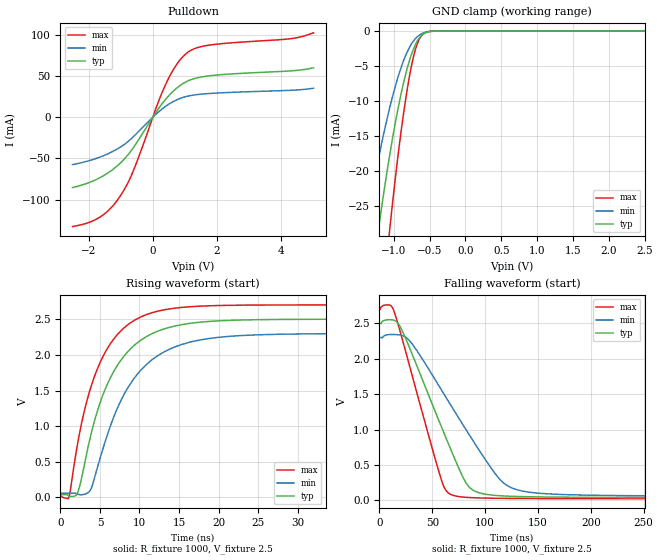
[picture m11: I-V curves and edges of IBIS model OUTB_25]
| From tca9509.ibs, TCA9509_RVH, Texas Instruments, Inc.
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[Model]   OUTB_25
Model_type  Open_drain
Enable   Active-High
Vref =   2.5
Rref =   1350
Cref =   50p
Vmeas =   1.25
| variable   typ   min   max
C_comp   2.86pF   1.87pF   3.29pF
| C_pulldown   2.91pF   2.13pF   4.07pF
| C_tri-state   2.86pF   1.87pF   3.29pF
[Temperature Range]   40   100   -40
| Ambient temperature   25   85   -40
[Voltage range]   2.5   2.3   2.7
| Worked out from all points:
|   slope of the pulldown table from 0 to 0.375 V, typ, clamps not added: 18.2 ohm
|   GND clamp passes 1 mA (typ) near -0.64 V on its own axis
|   rising waveform, R_fixture 1000, V_fixture 2.5: 20-80 % time 5.07ns typ, 5.86ns min, 4.5ns max; typ from 0.04 V to 2.5 V
|   falling waveform, R_fixture 1000, V_fixture 2.5: 20-80 % time 40.3ns typ, 56.6ns min, 29.6ns max; typ from 2.5 V to 0.04 V
[GND Clamp]
| OUTB_25
|   Voltage   I(typ)   I(min)   I(max)
-2.5V     -157.5mA   -111.4mA   -232.4mA
-1.4V     -43.18mA   -28.52mA   -67.74mA
-1.23V    -29.68mA   -19.14mA   -47.05mA
-1.205V   -27.84mA   -17.87mA   -44.2mA
-1.07V    -18.63mA   -11.58mA   -29.8mA
-1.05V    -17.38mA   -10.74mA   -27.82mA
-915mV    -9.842mA   -5.777mA   -15.78mA
-800mV    -4.902mA   -2.742mA   -7.638mA
-715mV    -2.35mA    -1.307mA   -3.298mA
-625mV    -778.3uA   -472.3uA   -845.3uA
-430mV    -20.32uA   -20.58uA   -8.486uA
2.5V      479.8pA    2.008nA    172pA
[Pulldown]
| OUTB_25
|   Voltage   I(typ)   I(min)   I(max)
-2.5V     -85.34mA   -57.53mA   -132.8mA
-1.635V   -73.16mA   -48.24mA   -121mA
-1.31V    -65.26mA   -42.78mA   -110.5mA
-1.01V    -55.58mA   -36.27mA   -95.43mA
-605mV    -36.88mA   -23.65mA   -64.87mA
145mV     8.615mA    5.278mA    15.87mA
405mV     22.03mA    13.37mA    40.34mA
730mV     34.94mA    20.85mA    63.42mA
1.045V    43.19mA    25.22mA    77.5mA
1.7V      50mA       28.64mA    87.22mA
4.255V    56.18mA    32.63mA    95.2mA
5V        60.04mA    35.23mA    102.5mA
[Ramp]
| OUTB_25
| variable   typ   min   max
dV/dt_r   1.49/5.07E-09   1.36/5.86E-09   1.63/4.50E-09
dV/dt_f   1.51/4.11E-08   1.37/5.75E-08   1.64/3.02E-08
R_load = 1000
[Rising Waveform]
| OUTB_25
R_fixture =   1000
C_fixture =   0
L_fixture =   0
V_fixture =   2.5
V_fixture_min = 2.3
V_fixture_max = 2.7
|   Time   V(typ)   V(min)   V(max)
0s        40.08mV    59.79mV    23.48mV
1.093ns   20.65mV    59.77mV    13.05mV
2.181ns   68.29mV    47.82mV    760.8mV
3.845ns   875.2mV    115.4mV    1.545V
6.213ns   1.654V     968.9mV    2.138V
7.941ns   1.968V     1.423V     2.368V
10.12ns   2.201V     1.778V     2.529V
16.13ns   2.438V     2.171V     2.672V
35.72ns   2.499V     2.297V     2.7V
317.1ns   2.5V       2.3V       2.7V
[Falling Waveform]
| OUTB_25
R_fixture =   1000
C_fixture =   0
L_fixture =   0
V_fixture =   2.5
V_fixture_min = 2.3
V_fixture_max = 2.7
|   Time   V(typ)   V(min)   V(max)
0s        2.5V       2.3V       2.7V
8.389ns   2.55V      2.34V      2.76V
13.45ns   2.545V     2.342V     2.685V
28.87ns   2.142V     2.248V     1.88V
57.54ns   1.079V     1.587V     342.1mV
66.76ns   745.8mV    1.363V     89.22mV
87.17ns   158.8mV    874.6mV    38.32mV
112.5ns   66.94mV    320.5mV    29.18mV
127.7ns   56.04mV    161.4mV    27.13mV
317.1ns   40.4mV     61.48mV    23.54mV
